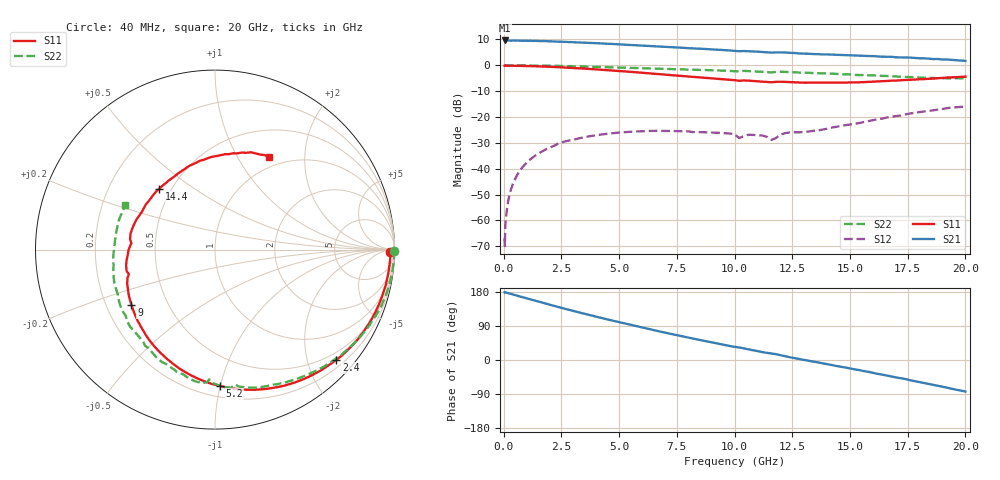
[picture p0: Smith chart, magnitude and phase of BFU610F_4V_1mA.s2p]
! Filename:  P:\Prog\Test\Noise\ATS_data\Testdata_Net\SplitFiles\BFU610_2W_A5_HighFreq_4V_1mA_D.s2p
! Date/Time: Wed 10/Aug/2011 16:57:34
! BFU610_2W_A5_HighFreq_4V_1mA_10mA_Bias1_R.s2p
! MDIF S-parameter v. bias file
! BFU610_2W_A5_HighFreq_4V_1mA_10mA
! Date/time Mon Aug 08 14:12:42 2011
! bias mode 1
! bias variable = I_out
! VAR bias_var= 1
! VAR V_out= 4.0000
! VAR I_out= 0.9950
! VAR V_in= 0.8451
! VAR I_in= 0.0070
! Device data file deembeded for feedlines and parallel
! Original file: \SplitFiles\BFU610_2W_A5_HighFreq_4V_1mA_R.s2p
! Feed-files: PR003V01_101208_Feed1.s2p, PR003V01_101208_Feed2.s2p
! Parallel-file: PR003V01_101208_Par.s2p
# MHz S MA R 50
!  Freq-MHz  S11-mag  S11-arg  S21-mag  S21-arg  S12-mag  S12-arg  S22-mag  S22-arg
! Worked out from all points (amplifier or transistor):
!   167 points, 40 MHz to 20 GHz, reference 50 ohm
!   highest |S21| = 9.6 dB at 40 MHz (marker M1)
!   |S21| within 3 dB of that: start of sweep to 8.025 GHz
!   unconditionally stable (mu >= 1): 7.943 GHz to end of sweep
!   at 550 MHz: K = -0.01, MSG = 26.2 dB, |S12| = -43.0 dB
!   at 4.2 GHz: K = 0.37, MSG = 17.6 dB, |S12| = -26.8 dB
!   at 20 GHz: K = 1.04, MAG = 7.5 dB, |S12| = -16.0 dB
!   S11 on the Smith chart (normalised r, x): 40 MHz: 68, -38; 2.4 GHz: 0.34, -2.55; 5.2 GHz: 0.28, -1.00; 9 GHz: 0.31, -0.28; 14.4 GHz: 0.43, +0.37; 20 GHz: 0.85, +1.37
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40  0.9778 -0.7  3.003 178.9  0.0004536 84.3  0.9977 -0.3
50  0.9751 -0.7  2.987 179.1  0.0003186 40.8  0.998 -0.5
60  0.9797 -1.0  2.995 178.3  0.0005617 103.3  0.9984 -0.5
80  0.9775 -1.4  3.002 178.2  0.0009205 89.7  0.9983 -0.7
220  0.9768 -3.9  2.99 176.0  0.002722 90.6  0.9982 -2.1
600  0.9721 -10.7  2.991 169.5  0.007792 85.8  0.9961 -5.7
1300  0.9559 -23.1  2.955 157.5  0.01706 76.0  0.9886 -12.3
2400  0.9133 -42.2  2.846 139.3  0.03097 61.8  0.9676 -22.6
3400  0.8637 -59.0  2.731 123.5  0.03984 49.5  0.9431 -31.3
4300  0.8135 -73.6  2.624 109.9  0.0462 39.7  0.9188 -38.6
5200  0.7601 -88.0  2.496 96.9  0.05068 31.0  0.894 -45.8
6800  0.6676 -113.0  2.285 74.7  0.05377 17.4  0.8514 -57.9
9000  0.5581 -146.5  2.023 46.8  0.05003 7.2  0.8 -74.0
10200  0.4987 -164.1  1.859 33.1  0.03913 1.0  0.7611 -81.5
10800  0.4957 -173.3  1.842 25.6  0.04498 9.2  0.7592 -87.4
11600  0.467 175.6  1.748 17.1  0.03595 11.4  0.7237 -92.5
12000  0.4793 169.3  1.769 12.5  0.04585 26.1  0.7468 -95.8
13400  0.46 146.9  1.643 -4.1  0.0539 24.1  0.704 -109.5
14400  0.4597 132.3  1.585 -15.7  0.0643 26.9  0.678 -119.9
16800  0.5023 99.5  1.452 -43.5  0.101 19.8  0.6136 -149.2
18400  0.5457 79.5  1.339 -63.2  0.131 7.5  0.5698 -174.8
20000  0.6007 59.7  1.21 -83.2  0.1592 -9.2  0.5573 153.8
